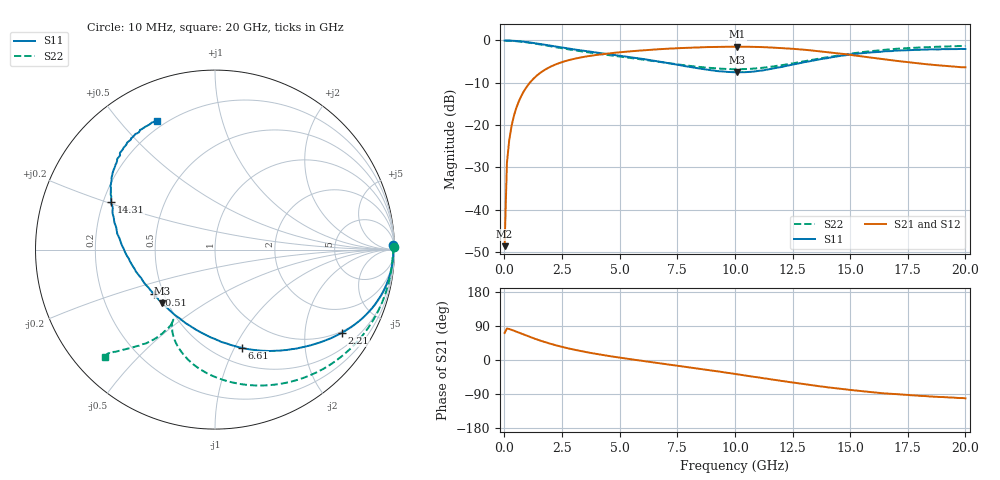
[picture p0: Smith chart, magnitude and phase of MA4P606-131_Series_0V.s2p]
! AWR Design Environment (9226) Thu Aug 19 15:24:37 2021
! Document = '0V'
! nPorts: 2, nXvals: 201
# GHz S DB R 50
!Freq DBS11 AngS11 DBS21 AngS21 DBS12 AngS12 DBS22 AngS22
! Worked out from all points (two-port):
!   201 points, 10 MHz to 20 GHz, reference 50 ohm
!   highest |S21| = -1.51 dB at 10.11 GHz (marker M1); lowest = -48.6 dB at 10 MHz (marker M2)
!   |S21| within 3 dB of the highest: 2.925 GHz to 16.5 GHz (13.58 GHz wide, 140 % of centre)
!   lowest |S11| = -7.6 dB at 10.11 GHz (marker M3), VSWR 2.44, Z = 23.4 - j17 ohm
!   |S11| at or under -10 dB: nowhere
!   |S22| runs from -6.8 to 0.0 dB; largest |S21 - S12| = 0.024
!   S11 on the Smith chart (normalised r, x): 10 MHz: 26, +77; 2.21 GHz: 0.95, -3.08; 6.61 GHz: 0.66, -1.07; 10.51 GHz: 0.44, -0.27; 14.31 GHz: 0.23, +0.21; 20 GHz: 0.17, +0.63
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0.01  -0.07 1.3  -48.62 71.5  -47.29 67.4  -0.04 0.9
0.11  -0.06 -2.1  -29.04 83.1  -29.07 83.3  -0.09 -3.8
0.21  -0.07 -3.9  -23.58 81.7  -23.57 82.0  -0.10 -7.3
0.41  -0.12 -7.4  -17.92 77.4  -17.92 77.5  -0.16 -14.1
0.71  -0.25 -12.6  -13.41 70.2  -13.41 70.3  -0.31 -24.0
1.11  -0.52 -19.0  -9.99 60.8  -9.98 61.0  -0.59 -36.5
1.61  -0.93 -26.0  -7.48 50.1  -7.48 50.5  -1.03 -50.4
2.21  -1.46 -33.3  -5.73 39.2  -5.72 39.7  -1.61 -64.3
3.41  -2.45 -45.0  -3.96 22.5  -3.93 23.2  -2.67 -84.8
4.81  -3.49 -57.2  -2.93 8.1  -2.91 8.8  -3.70 -100.4
6.61  -4.93 -74.9  -2.14 -7.5  -2.10 -6.6  -5.01 -112.9
6.71  -5.02 -76.0  -2.11 -8.3  -2.06 -7.4  -5.08 -113.5
8.41  -6.62 -100.1  -1.67 -22.7  -1.63 -21.6  -6.26 -119.6
10.01  -7.56 -132.1  -1.51 -36.9  -1.46 -35.5  -6.85 -120.8
10.11  -7.57 -134.4  -1.51 -37.7  -1.46 -36.4  -6.84 -120.7
10.51  -7.52 -143.5  -1.52 -41.3  -1.47 -39.9  -6.79 -120.6
11.91  -6.40 -172.3  -1.80 -54.2  -1.71 -52.6  -5.98 -120.6
13.41  -4.76 165.4  -2.44 -66.9  -2.33 -65.7  -4.56 -123.6
14.31  -3.93 155.4  -2.98 -74.0  -2.86 -72.8  -3.72 -126.5
16.71  -2.57 136.0  -4.65 -89.0  -4.61 -87.9  -2.15 -133.7
19.01  -2.08 122.1  -5.97 -97.7  -6.09 -97.3  -1.50 -135.9
20  -2.06 114.3  -6.37 -101.1  -6.57 -100.0  -1.34 -135.5
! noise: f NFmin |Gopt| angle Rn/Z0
0.01  0  1  0  2e-20
2.21  0  1  0  2e-20
4.41  0  1  0  2e-20
6.61  0  1  0  2e-20
8.81  0  1  0  2e-20
11.11  0  1  0  2e-20
13.31  0  1  0  2e-20
15.51  0  1  0  2e-20
17.71  0  1  0  2e-20
20  0  1  0  2e-20
